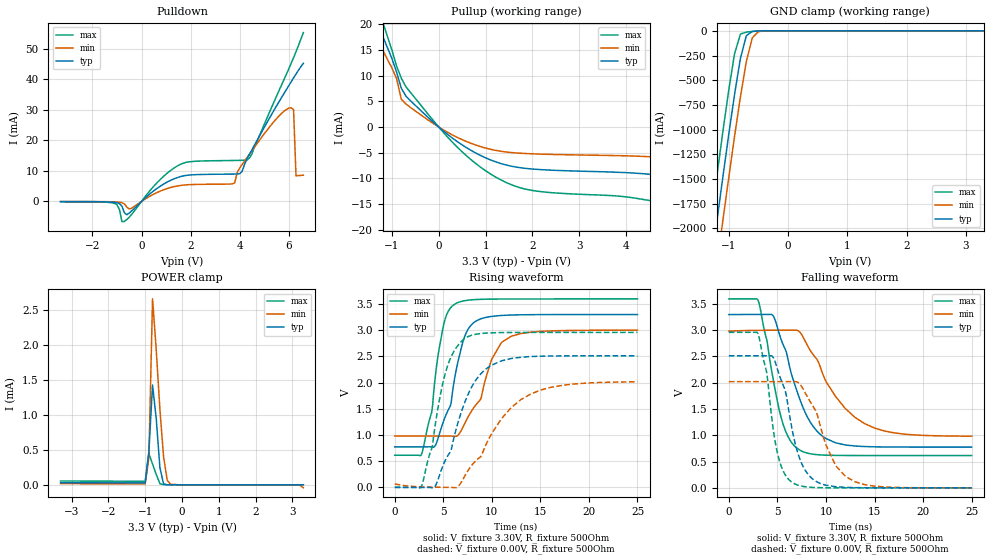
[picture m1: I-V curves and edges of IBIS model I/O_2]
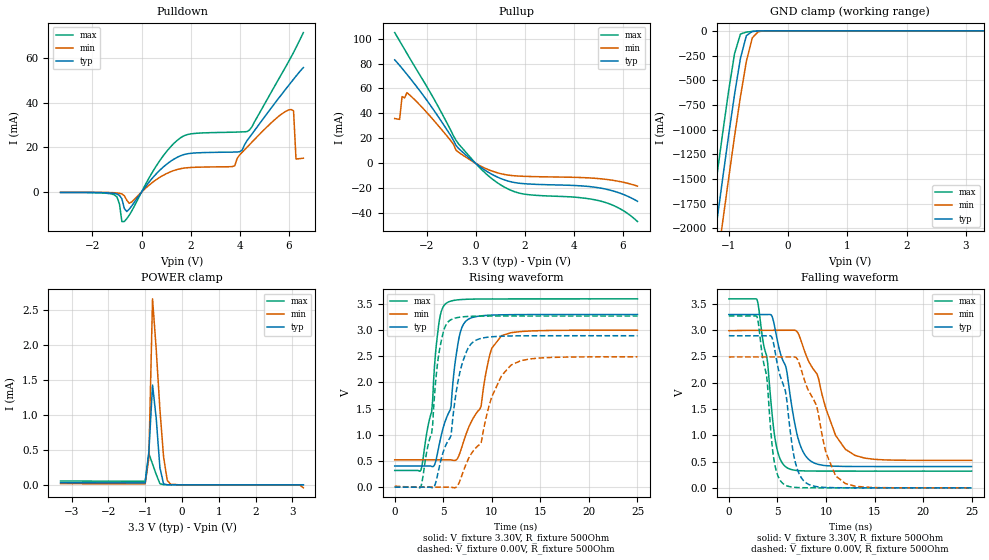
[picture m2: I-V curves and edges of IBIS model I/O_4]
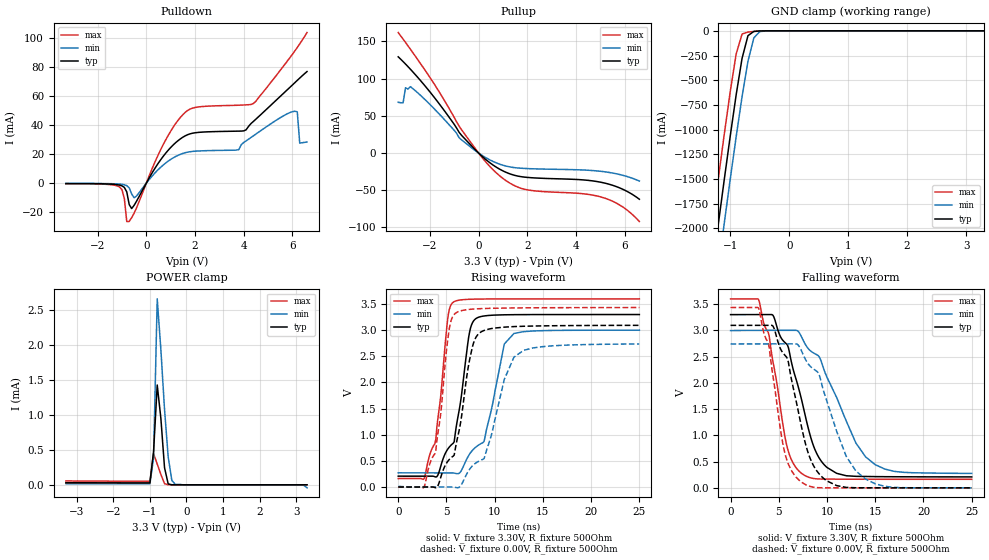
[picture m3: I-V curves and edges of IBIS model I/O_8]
[IBIS Ver]   3.2
[File Name]   lm3s5749_lqfp_v0p1.ibs
[File Rev]   0.1
[Date]   02/22/2010
[Source]   From silicon level SPICE simulations at Texas Instruments
[Notes]   Initial Release of IBIS model
   LM3S5749, Revision A0, 100 LQFP
[Disclaimer] Texas Instruments Confidential - Advance Product Information
   < Software License Agreement >
  Texas Instruments (TI) is supplying this software for use solely and
  exclusively on TI's Stellaris Family of microcontroller products.
  The software is owned by TI and/or its suppliers, and is protected under
  applicable copyright laws.  All rights are reserved.  Any use in violation
  of the foregoing restrictions may subject the user to criminal sanctions
  under applicable laws, as well as to civil liability for the breach of the
  terms and conditions of this license.
  THIS SOFTWARE IS PROVIDED "AS IS".  NO WARRANTIES, WHETHER EXPRESS, IMPLIED
  OR STATUTORY, INCLUDING, BUT NOT LIMITED TO, IMPLIED WARRANTIES OF
  MERCHANTABILITY AND FITNESS FOR A PARTICULAR PURPOSE APPLY TO THIS SOFTWARE.
  LMI SHALL NOT, IN ANY CIRCUMSTANCES, BE LIABLE FOR SPECIAL, INCIDENTAL, OR
  CONSEQUENTIAL DAMAGES, FOR ANY REASON WHATSOEVER.
[Copyright]   Copyright (c) 2010 Texas Instruments.  All rights reserved.
[Component]   LM3S5749 100LQFP
[Manufacturer]  Texas Instruments
[Package]
| 100-pin LQFP
| variable   typ   min   max
R_pkg   125.000m   98.000m   152.000m
L_pkg   7.745nH   6.720nH   8.770nH
C_pkg   0.745pF   0.660pF   0.830pF
[Pin]  signal_name   model_name
   1   PE7_ADC0   ProgBuff
   2   PE6_ADC1   ProgBuff
   3   VDDA   POWER
   4   GNDA   GND
   5   PE5_ADC2   ProgBuff
   6   PE4_ADC3   ProgBuff
   7   LDO   POWER
   8   VDD   POWER
   9   GND   GND
  10   PD0_CAN0Rx   ProgBuff
  11   PD1_CAN0Tx   ProgBuff
  12   PD2_U1Rx   ProgBuff
  13   PD3_U1Tx   ProgBuff
  14   VDD25   POWER
  15   GND   GND
  16   PG3_Fault2   ProgBuff
  17   PG2_Fault0   ProgBuff
  18   PG1_PWM1   ProgBuff
  19   PG0_PWM0   ProgBuff
  20   VDD   POWER
  21   GND   GND
  22   PC7_CCP4   ProgBuff
  23   PC6_CCP3   ProgBuff
  24   PC5   ProgBuff
  25   PC4_CCP2   ProgBuff
  26   PA0_U0Rx   ProgBuff
  27   PA1_U0Tx   ProgBuff
  28   PA2_SSI0Clk   ProgBuff
  29   PA3_SSI0Fss   ProgBuff
  30   PA4_SSI0Rx   ProgBuff
  31   PA5_SSI0Tx   ProgBuff
  32   VDD   POWER
  33   GND   GND
  34   PA6_I2C1SCL   ProgBuff
  35   PA7_I2C1SDA   ProgBuff
  36   PG7_PWM7   ProgBuff
  37   PG6_PWM6   ProgBuff
  38   VDD25   POWER
  39   GND   GND
  40   PG5_IDX0   ProgBuff
  41   PG4_Fault1   ProgBuff
  42   PF7_PhB0   ProgBuff
  43   PF6_PhA0   ProgBuff
  44   VDD   POWER
  45   GND   GND
  46   PF5_C1o   ProgBuff
  47   PF0_CAN1Rx   ProgBuff
  48   OSC0   NC
  49   OSC1   NC
  50   WAKE   NC
  51   HIB   NC
  52   XOSC0   NC
  53   XOSC1   NC
  54   GND   GND
  55   VBAT   POWER
  56   VDD   POWER
  57   GND   GND
  58   PF4_C0o   ProgBuff
  59   PF3_PWM5   ProgBuff
  60   PF2_PWM4   ProgBuff
  61   PF1_CAN1Tx   ProgBuff
  62   VDD25   POWER
  63   GND   GND
  64   RST   NC
  65   PB3_I2C0SDA   ProgBuff
  66   PB0_CCP0   ProgBuff
  67   PB1_CCP1   ProgBuff
  68   VDD   POWER
  69   GND   GND
  70   USB0DM   NC
  71   USB0DP   NC
  72   PB2_I2C0SCL   ProgBuff
  73   USB0RBIAS   NC
  74   PE0_SSI1Clk   ProgBuff
  75   PE1_SSI1Fss   ProgBuff
  76   PH4_USB0PFLT   ProgBuff
  77   PC3_TDO_SWO   ProgBuff
  78   PC2_TDI   ProgBuff
  79   PC1_TMS_SWDIO   ProgBuff
  80   PC0_TCK_SWCLK   ProgBuff
  81   VDD   POWER
  82   GND   GND
  83   PH3_USB0EPEN   ProgBuff
  84   PH2_Fault3   ProgBuff
  85   PH1_PWM3   ProgBuff
  86   PH0_PWM2   ProgBuff
  87   GND   GND
  88   VDD25   POWER
  89   PB7_NMI   ProgBuff
  90   PB6   ProgBuff
  91   PB5   ProgBuff
  92   PB4   ProgBuff
  93   VDD   POWER
  94   GND   GND
  95   PE2_SSI1Rx   ProgBuff
  96   PE3_SSI1Tx   ProgBuff
  97   PD4_ADC7   ProgBuff
  98   PD5_ADC6   ProgBuff
  99   PD6_ADC5   ProgBuff
 100   PD7_ADC4   ProgBuff
[Model Selector]   ProgBuff
I/O_2   2 mA buffer without slew rate control
I/O_4   4 mA buffer without slew rate control
I/O_8   8 mA buffer without slew rate control
I/O_8S   8 mA buffer with slew rate control
OD_I/O_2   open-drain 2 mA buffer without slew rate control
OD_I/O_4   open-drain 4 mA buffer without slew rate control
OD_I/O_8   open-drain 8 mA buffer without slew rate control
OD_I/O_8S   open-drain 8 mA buffer with slew rate control
WPU_I/O_2   weak pullup 2 mA buffer without slew rate control
WPU_I/O_4   weak pullup 4 mA buffer without slew rate control
WPU_I/O_8   weak pullup 8 mA buffer without slew rate control
WPU_I/O_8S   weak pullup 8 mA buffer with slew rate control
WPD_I/O_2   weak pulldown 2 mA buffer without slew rate control
WPD_I/O_4   weak pulldown 4 mA buffer without slew rate control
WPD_I/O_8   weak pulldown 8 mA buffer without slew rate control
WPD_I/O_8S   weak pulldown 8 mA buffer with slew rate control
| Models and submodels in the file (16): I/O_2 (I/O), I/O_4 (I/O), I/O_8 (I/O), I/O_8S (I/O), OD_I/O_2 (I/O_open_drain), OD_I/O_4 (I/O_open_drain), OD_I/O_8 (I/O_open_drain), OD_I/O_8S (I/O_open_drain), WPU_I/O_2 (I/O), WPU_I/O_4 (I/O), WPU_I/O_8 (I/O), WPU_I/O_8S (I/O), WPD_I/O_2 (I/O), WPD_I/O_4 (I/O), WPD_I/O_8 (I/O), WPD_I/O_8S (I/O)
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[Model]   I/O_2
Model_type   I/O
Vinl = 1.26
Vinh = 2.04
Vmeas = 1.65
| variable   typ   min   max
C_comp   9.739pF   9.739pF   9.803pF
[Model Spec]
Vinh+   1.91   1.78   2.04
Vinh-   1.90   1.76   2.03
Vinl+   1.40   1.27   1.54
Vinl-   1.39   1.26   1.53
| variable   typ   min   max
[Temperature Range]  25   85   -40
[Voltage Range]   3.3V   3.0V   3.6V
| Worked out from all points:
|   slope of the pulldown table from 0 to 0.495 V, typ, clamps not added: 143 ohm
|   slope of the pullup table from 0 to 0.495 V, typ, clamps not added: 143 ohm
|   GND clamp passes 1 mA (typ) near -0.48 V on its own axis
|   POWER clamp passes 1 mA (typ) near -0.71 V on its own axis
|   falling waveform, V_fixture 3.30V, R_fixture 500Ohm: 20-80 % time 2.85ns typ, 4.24ns min, 1.93ns max; typ from 3.29 V to 0.774 V
|   rising waveform, V_fixture 3.30V, R_fixture 500Ohm: 20-80 % time 1.99ns typ, 2.79ns min, 1.46ns max; typ from 0.774 V to 3.3 V
|   falling waveform, V_fixture 0.00V, R_fixture 500Ohm: 20-80 % time 1.94ns typ, 2.63ns min, 1.43ns max; typ from 2.51 V to 0 V
|   rising waveform, V_fixture 0.00V, R_fixture 500Ohm: 20-80 % time 3.04ns typ, 4.58ns min, 2ns max; typ from 0.005 V to 2.51 V
[Pulldown]
|  Voltage   I(typ)   I(min)   I(max)
-3.3V     -64.15uA   -36.41uA   -91.13uA
-1.1V     -318.3uA   -146.9uA   -641.8uA
-700mV    -3.678mA   -803.7uA   -6.582mA
-500mV    -3.814mA   -2.5mA     -5.165mA
1.6V      8.164mA    5.256mA    12.21mA
3.8V      8.971mA    6.071mA    13.44mA
4.1V      9.802mA    12.05mA    13.49mA
4.3V      13.99mA    14.33mA    13.56mA
6.1V      39.18mA    30.7mA     45.23mA
6.2V      40.48mA    30.1mA     47.14mA
6.3V      41.75mA    8.417mA    49.11mA
6.6V      45.28mA    8.602mA    55.36mA
[Pullup]
|  Voltage   I(typ)   I(min)   I(max)
-3.3V     58.84mA    18.65mA    75.09mA
-1.5V     24.39mA    20.24mA    28.75mA
-1.3V     20.01mA    16.77mA    23.31mA
-1.2V     17.8mA     15.03mA    20.55mA
-900mV    10.69mA    9.417mA    11.87mA
-800mV    7.564mA    5.426mA    9.531mA
-700mV    6.024mA    4.488mA    7.83mA
500mV     -3.489mA   -2.46mA    -4.836mA
1.5V      -7.533mA   -4.924mA   -11.05mA
5V        -9.793mA   -6.102mA   -15.25mA
6V        -12.34mA   -7.492mA   -19.35mA
6.6V      -15.07mA   -8.994mA   -23.96mA
[GND Clamp]
|  Voltage   I(typ)   I(min)   I(max)
-3.3V     -11.73A    -12.14A    -11.32A
-1.4V     -2.85A     -3.29A     -2.391A
-1.3V     -2.393A    -2.835A    -1.933A
-1.2V     -1.942A    -2.383A    -1.481A
-1.1V     -1.496A    -1.937A    -1.038A
-1V       -1.061A    -1.498A    -612.1mA
-900mV    -646.5mA   -1.071A    -233.9mA
-800mV    -278.2mA   -665.9mA   -32.18mA
-700mV    -49.12mA   -307.7mA   -12.49mA
-600mV    -5.764mA   -70.86mA   -6.504mA
-500mV    -1.206mA   -8.171mA   -2.256mA
3.3V      2.312nA    3.21uA     471pA
[POWER Clamp]
|  Voltage   I(typ)   I(min)   I(max)
-3.3V     29.71uA    15.87uA    54.94uA
-1V       27.67uA    14.78uA    51.22uA
-900mV    475.3uA    385.2uA    446.8uA
-800mV    1.43mA     2.664mA    297.3uA
-700mV    950.8uA    1.937mA    147.8uA
-600mV    244.5uA    1.079mA    15.75uA
-500mV    13.05uA    399.9uA    1.307uA
-400mV    328.8nA    62.11uA    58.57nA
-300mV    10.28nA    3.21uA     1.749nA
3.1V      1.297nA    -118nA     134.9pA
3.2V      1.2nA      -2.426uA   122pA
3.3V      -118pA     -43.75uA   108.5pA
[Ramp]
| variable   typ   min   max
dV/dt_f   1.51/2.85n   1.20/4.24n   1.79/1.93n
dV/dt_r   1.50/3.04n   1.17/4.58n   1.77/2.00n
R_load = 500Ohm
[Falling Waveform]
V_fixture = 3.30V
V_fixture_min = 3.00V
V_fixture_max = 3.60V
R_fixture = 500Ohm
|   Time   V(typ)   V(min)   V(max)
0s        3.293V     2.978V     3.591V
3ns       3.295V     2.993V     3.57V
4.5ns     3.284V     2.995V     2.131V
5.4ns     2.81V      2.996V     1.328V
7.2ns     1.741V     2.978V     729.6mV
8.4ns     1.246V     2.607V     647.5mV
9.7ns     974.5mV    2.152V     623.1mV
12ns      815mV      1.507V     615.1mV
14ns      784.7mV    1.219V     614.3mV
25ns      774.3mV    981.9mV    614.1mV
[Rising Waveform]
V_fixture = 3.30V
V_fixture_min = 3.00V
V_fixture_max = 3.60V
R_fixture = 500Ohm
|   Time   V(typ)   V(min)   V(max)
0s        774.3mV    980.2mV    614.1mV
2.8ns     774.3mV    980mV      649.9mV
3.8ns     770.2mV    980mV      1.426V
5ns       1.249V     979.9mV    3.068V
5.8ns     1.6V       979.6mV    3.434V
6.2ns     2.111V     973mV      3.496V
7.9ns     3.101V     1.453V     3.576V
10ns      3.261V     2.448V     3.59V
12ns      3.287V     2.883V     3.592V
25ns      3.296V     2.998V     3.594V
[Falling Waveform]
V_fixture = 0.00V
V_fixture_min = 0.00V
V_fixture_max = 0.00V
R_fixture = 500Ohm
|   Time   V(typ)   V(min)   V(max)
0s        2.51V      2.018V     2.956V
3ns       2.51V      2.018V     2.933V
3.9ns     2.51V      2.018V     2.19V
5ns       2.258V     2.018V     667.7mV
5.9ns     1.774V     2.018V     221mV
6.6ns     1.032V     2.019V     94.37mV
8.4ns     206.6mV    1.631V     11.33mV
11ns      21.52mV    421.7mV    712.2uV
12ns      9.312mV    217.6mV    301.3uV
25ns      30.04uV    131.8uV    20.33uV
[Rising Waveform]
V_fixture = 0.00V
V_fixture_min = 0.00V
V_fixture_max = 0.00V
R_fixture = 500Ohm
|   Time   V(typ)   V(min)   V(max)
0s        4.944mV    67.69mV    205.5uV
2.8ns     491.8uV    11.6mV     38.62mV
4.1ns     7.126mV    5.277mV    1.099V
5.3ns     550.3mV    2.605mV    2.232V
6.4ns     1.16V      2.696mV    2.679V
7.3ns     1.663V     245.8mV    2.849V
9.7ns     2.299V     928mV      2.945V
12ns      2.458V     1.522V     2.954V
14ns      2.495V     1.781V     2.955V
25ns      2.51V      2.014V     2.956V
[Model]   I/O_4
Model_type   I/O
Vinl = 1.26
Vinh = 2.04
Vmeas = 1.65
| variable   typ   min   max
C_comp   9.739pF   9.739pF   9.803pF
[Model Spec]
Vinh+   1.91   1.78   2.04
Vinh-   1.90   1.76   2.03
Vinl+   1.40   1.27   1.54
Vinl-   1.39   1.26   1.53
| variable   typ   min   max
[Temperature Range]  25   85   -40
[Voltage Range]   3.3V   3.0V   3.6V
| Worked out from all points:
|   slope of the pulldown table from 0 to 0.495 V, typ, clamps not added: 71.5 ohm
|   slope of the pullup table from 0 to 0.495 V, typ, clamps not added: 71.6 ohm
|   GND clamp passes 1 mA (typ) near -0.48 V on its own axis
|   POWER clamp passes 1 mA (typ) near -0.71 V on its own axis
|   falling waveform, V_fixture 3.30V, R_fixture 500Ohm: 20-80 % time 1.98ns typ, 2.95ns min, 1.33ns max; typ from 3.3 V to 0.405 V
|   rising waveform, V_fixture 3.30V, R_fixture 500Ohm: 20-80 % time 1.71ns typ, 2.4ns min, 1.18ns max; typ from 0.405 V to 3.3 V
|   falling waveform, V_fixture 0.00V, R_fixture 500Ohm: 20-80 % time 1.7ns typ, 2.49ns min, 1.18ns max; typ from 2.89 V to 0 V
|   rising waveform, V_fixture 0.00V, R_fixture 500Ohm: 20-80 % time 2.03ns typ, 3.15ns min, 1.33ns max; typ from 0 V to 2.89 V
[Pulldown]
|  Voltage   I(typ)   I(min)   I(max)
-3.3V     -128.3uA   -72.81uA   -182.3uA
-1.1V     -636.5uA   -293.8uA   -1.284mA
-700mV    -7.355mA   -1.607mA   -13.16mA
-500mV    -7.628mA   -5mA       -10.33mA
700mV     9.309mA    6.304mA    13.37mA
1.6V      16.33mA    10.51mA    24.41mA
3.8V      17.94mA    11.77mA    26.87mA
4.4V      24.49mA    21.21mA    27.8mA
6V        47.81mA    36.8mA     58.52mA
6.2V      50.6mA     36.46mA    62.59mA
6.3V      51.97mA    14.83mA    64.73mA
6.6V      55.82mA    15.21mA    71.49mA
[Pullup]
|  Voltage   I(typ)   I(min)   I(max)
-3.3V     82.94mA    35.91mA    104.8mA
-3.1V     78.46mA    35.23mA    98.11mA
-3V       76.12mA    53.49mA    94.75mA
-2.9V     73.74mA    52.42mA    91.4mA
-2.8V     71.31mA    56.64mA    88.05mA
-1.6V     39.56mA    31.96mA    48.08mA
-800mV    14.33mA    10.47mA    18.43mA
700mV     -9.22mA    -6.424mA   -12.9mA
1.9V      -16.2mA    -10.35mA   -24.39mA
5.2V      -20.25mA   -12.6mA    -30.84mA
5.9V      -24.02mA   -14.69mA   -36.54mA
6.6V      -30.45mA   -18.28mA   -46.68mA
[GND Clamp]
|  Voltage   I(typ)   I(min)   I(max)
-3.3V     -11.73A    -12.14A    -11.32A
-1.4V     -2.85A     -3.29A     -2.391A
-1.3V     -2.393A    -2.835A    -1.933A
-1.2V     -1.942A    -2.383A    -1.481A
-1.1V     -1.496A    -1.937A    -1.038A
-1V       -1.061A    -1.498A    -612.1mA
-900mV    -646.5mA   -1.071A    -233.9mA
-800mV    -278.2mA   -665.9mA   -32.18mA
-700mV    -49.12mA   -307.7mA   -12.49mA
-600mV    -5.764mA   -70.86mA   -6.504mA
-500mV    -1.206mA   -8.171mA   -2.256mA
3.3V      2.312nA    3.21uA     471pA
[POWER Clamp]
|  Voltage   I(typ)   I(min)   I(max)
-3.3V     29.71uA    15.87uA    54.94uA
-1V       27.67uA    14.78uA    51.22uA
-900mV    475.3uA    385.2uA    446.8uA
-800mV    1.43mA     2.664mA    297.3uA
-700mV    950.8uA    1.937mA    147.8uA
-600mV    244.5uA    1.079mA    15.75uA
-500mV    13.05uA    399.9uA    1.307uA
-400mV    328.8nA    62.11uA    58.57nA
-300mV    10.28nA    3.21uA     1.749nA
3.1V      1.297nA    -118nA     134.9pA
3.2V      1.2nA      -2.426uA   122pA
3.3V      -118pA     -43.75uA   108.5pA
[Ramp]
| variable   typ   min   max
dV/dt_f   1.73/1.98n   1.48/2.95n   1.97/1.33n
dV/dt_r   1.74/2.03n   1.48/3.15n   1.96/1.33n
R_load = 500Ohm
[Falling Waveform]
V_fixture = 3.30V
V_fixture_min = 3.00V
V_fixture_max = 3.60V
R_fixture = 500Ohm
|   Time   V(typ)   V(min)   V(max)
0s        3.297V     2.99V      3.595V
2.9ns     3.297V     2.997V     3.584V
4ns       3.298V     2.998V     2.371V
4.8ns     2.99V      2.998V     887.6mV
5.9ns     2.286V     2.998V     394.2mV
7.1ns     961.8mV    2.952V     328.8mV
8.6ns     491.2mV    2.287V     319.7mV
11ns      411.2mV    995.1mV    318.6mV
13ns      406.3mV    617mV      318.5mV
25ns      405.4mV    522.4mV    318.5mV
[Rising Waveform]
V_fixture = 3.30V
V_fixture_min = 3.00V
V_fixture_max = 3.60V
R_fixture = 500Ohm
|   Time   V(typ)   V(min)   V(max)
0s        405.4mV    522.4mV    318.5mV
2.7ns     405.4mV    522.4mV    325.5mV
3.8ns     396.2mV    522.4mV    1.436V
4.6ns     825.6mV    522.4mV    3.19V
5.3ns     1.309V     522.4mV    3.512V
5.8ns     1.54V      520.4mV    3.555V
6.7ns     2.919V     646.8mV    3.582V
7.6ns     3.21V      1.134V     3.59V
11ns      3.293V     2.895V     3.596V
25ns      3.298V     2.999V     3.597V
[Falling Waveform]
V_fixture = 0.00V
V_fixture_min = 0.00V
V_fixture_max = 0.00V
R_fixture = 500Ohm
|   Time   V(typ)   V(min)   V(max)
0s        2.893V     2.49V      3.27V
2.9ns     2.893V     2.491V     3.258V
3.9ns     2.893V     2.491V     2.117V
4.6ns     2.755V     2.491V     588.5mV
5.7ns     1.917V     2.491V     64.29mV
6.8ns     521.4mV    2.49V      9.46mV
8.1ns     77.91mV    1.893V     1.44mV
10ns      7.517mV    669mV      209.9uV
12ns      1.014mV    81.45mV    73.19uV
25ns      18.39uV    38.9uV     11.44uV
[Rising Waveform]
V_fixture = 0.00V
V_fixture_min = 0.00V
V_fixture_max = 0.00V
R_fixture = 500Ohm
|   Time   V(typ)   V(min)   V(max)
0s        491.5uV    19.4mV     17.4uV
2.7ns     45.46uV    2.137mV    9.061mV
3.8ns     -8.433mV   973.8uV    1.029V
4.6ns     394.1mV    558.2uV    2.609V
5.7ns     943.7mV    269.7uV    3.188V
6.8ns     2.261V     163.8mV    3.25V
8.3ns     2.8V       740.2mV    3.266V
10ns      2.873V     1.728V     3.269V
12ns      2.889V     2.335V     3.269V
25ns      2.893V     2.49V      3.27V
[Model]   I/O_8
Model_type   I/O
Vinl = 1.26
Vinh = 2.04
Vmeas = 1.65
| variable   typ   min   max
C_comp   9.739pF   9.739pF   9.803pF
[Model Spec]
Vinh+   1.91   1.78   2.04
Vinh-   1.90   1.76   2.03
Vinl+   1.40   1.27   1.54
Vinl-   1.39   1.26   1.53
| variable   typ   min   max
[Temperature Range]  25   85   -40
[Voltage Range]   3.3V   3.0V   3.6V
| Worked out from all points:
|   slope of the pulldown table from 0 to 0.495 V, typ, clamps not added: 35.8 ohm
|   slope of the pullup table from 0 to 0.495 V, typ, clamps not added: 35.8 ohm
|   GND clamp passes 1 mA (typ) near -0.48 V on its own axis
|   POWER clamp passes 1 mA (typ) near -0.71 V on its own axis
|   falling waveform, V_fixture 3.30V, R_fixture 500Ohm: 20-80 % time 2.57ns typ, 3.82ns min, 1.8ns max; typ from 3.3 V to 0.208 V
|   rising waveform, V_fixture 3.30V, R_fixture 500Ohm: 20-80 % time 1.54ns typ, 2.24ns min, 1.14ns max; typ from 0.208 V to 3.3 V
|   falling waveform, V_fixture 0.00V, R_fixture 500Ohm: 20-80 % time 2.29ns typ, 3.1ns min, 1.68ns max; typ from 3.09 V to 0 V
|   rising waveform, V_fixture 0.00V, R_fixture 500Ohm: 20-80 % time 1.64ns typ, 2.39ns min, 1.21ns max; typ from 0 V to 3.09 V
[Pulldown]
|  Voltage   I(typ)   I(min)   I(max)
-3.3V     -256.6uA   -145.6uA   -364.5uA
-1.1V     -1.273mA   -587.5uA   -2.567mA
-700mV    -14.71mA   -3.215mA   -26.33mA
-500mV    -15.26mA   -10mA      -20.66mA
600mV     16.36mA    11.13mA    23.41mA
1.5V      31.68mA    20.52mA    47.2mA
3.8V      35.88mA    23.15mA    53.74mA
4.4V      42.6mA     32.69mA    54.98mA
6.1V      69.26mA    49.6mA     91.12mA
6.2V      70.84mA    49.17mA    93.51mA
6.3V      72.42mA    27.66mA    95.98mA
6.6V      76.89mA    28.41mA    103.8mA
[Pullup]
|  Voltage   I(typ)   I(min)   I(max)
-3.3V     129.3mA    68.2mA     161.9mA
-3.1V     122.9mA    67.41mA    153.1mA
-3V       119.6mA    87.83mA    148.7mA
-2.8V     112.7mA    89.21mA    139.6mA
-1.8V     73.98mA    58.72mA    91.66mA
-700mV    23.83mA    17.72mA    31.29mA
300mV     -8.845mA   -6.303mA   -12.15mA
1V        -23.99mA   -16.37mA   -34.1mA
2V        -32.73mA   -20.87mA   -49.46mA
5.1V      -39.81mA   -24.88mA   -59.77mA
5.9V      -48.4mA    -29.75mA   -72.06mA
6.6V      -62.06mA   -37.61mA   -92.08mA
[GND Clamp]
|  Voltage   I(typ)   I(min)   I(max)
-3.3V     -11.73A    -12.14A    -11.32A
-1.4V     -2.85A     -3.29A     -2.391A
-1.3V     -2.393A    -2.835A    -1.933A
-1.2V     -1.942A    -2.383A    -1.481A
-1.1V     -1.496A    -1.937A    -1.038A
-1V       -1.061A    -1.498A    -612.1mA
-900mV    -646.5mA   -1.071A    -233.9mA
-800mV    -278.2mA   -665.9mA   -32.18mA
-700mV    -49.12mA   -307.7mA   -12.49mA
-600mV    -5.764mA   -70.86mA   -6.504mA
-500mV    -1.206mA   -8.171mA   -2.256mA
3.3V      2.312nA    3.21uA     471pA
[POWER Clamp]
|  Voltage   I(typ)   I(min)   I(max)
-3.3V     29.71uA    15.87uA    54.94uA
-1V       27.67uA    14.78uA    51.22uA
-900mV    475.3uA    385.2uA    446.8uA
-800mV    1.43mA     2.664mA    297.3uA
-700mV    950.8uA    1.937mA    147.8uA
-600mV    244.5uA    1.079mA    15.75uA
-500mV    13.05uA    399.9uA    1.307uA
-400mV    328.8nA    62.11uA    58.57nA
-300mV    10.28nA    3.21uA     1.749nA
3.1V      1.297nA    -118nA     134.9pA
3.2V      1.2nA      -2.426uA   122pA
3.3V      -118pA     -43.75uA   108.5pA
[Ramp]
| variable   typ   min   max
dV/dt_f   1.85/2.57n   1.63/3.82n   2.06/1.80n
dV/dt_r   1.86/1.64n   1.63/2.39n   2.06/1.21n
R_load = 500Ohm
[Falling Waveform]
V_fixture = 3.30V
V_fixture_min = 3.00V
V_fixture_max = 3.60V
R_fixture = 500Ohm
|   Time   V(typ)   V(min)   V(max)
0s        3.298V     2.994V     3.597V
2.9ns     3.298V     2.998V     3.588V
4ns       3.298V     2.998V     2.898V
5.9ns     2.717V     2.999V     754.8mV
7.4ns     1.65V      2.859V     271.3mV
8.6ns     799.3mV    2.568V     178.4mV
9.8ns     422.5mV    2.192V     166.9mV
13ns      219mV      852mV      163.9mV
15ns      214mV      441.3mV    163.3mV
25ns      208.2mV    274.5mV    162.3mV
[Rising Waveform]
V_fixture = 3.30V
V_fixture_min = 3.00V
V_fixture_max = 3.60V
R_fixture = 500Ohm
|   Time   V(typ)   V(min)   V(max)
0s        207.6mV    271.4mV    162.2mV
2.7ns     207.4mV    270.4mV    165.3mV
3.9ns     191.8mV    270.1mV    914mV
5.1ns     714.8mV    269.9mV    3.171V
5.7ns     836.9mV    269.3mV    3.533V
7.4ns     2.965V     630.1mV    3.591V
8.1ns     3.227V     771.5mV    3.594V
11ns      3.294V     2.736V     3.597V
12ns      3.296V     2.937V     3.597V
25ns      3.299V     2.999V     3.598V
[Falling Waveform]
V_fixture = 0.00V
V_fixture_min = 0.00V
V_fixture_max = 0.00V
R_fixture = 500Ohm
|   Time   V(typ)   V(min)   V(max)
0s        3.093V     2.739V     3.433V
2.9ns     3.093V     2.74V      3.423V
4ns       3.094V     2.741V     2.68V
5.6ns     2.532V     2.741V     685.6mV
7.3ns     1.21V      2.629V     116.7mV
8.2ns     586.3mV    2.327V     30.35mV
9.4ns     222.8mV    2.013V     1.741mV
12ns      7.855mV    597.6mV    107.7uV
14ns      1.389mV    166.7mV    70.3uV
25ns      37.48uV    42.83uV    16.46uV
[Rising Waveform]
V_fixture = 0.00V
V_fixture_min = 0.00V
V_fixture_max = 0.00V
R_fixture = 500Ohm
|   Time   V(typ)   V(min)   V(max)
0s        365.8uV    12.24mV    108.2uV
2.7ns     122.3uV    1.727mV    4.268mV
3.9ns     -14.91mV   677.3uV    699.6mV
5.2ns     506.2mV    277.7uV    2.901V
5.9ns     711.2mV    -6.26mV    3.319V
7.5ns     2.521V     363.7mV    3.399V
8.5ns     2.956V     507.8mV    3.411V
9ns       3.001V     598.7mV    3.414V
12ns      3.068V     2.484V     3.425V
25ns      3.092V     2.736V     3.432V
